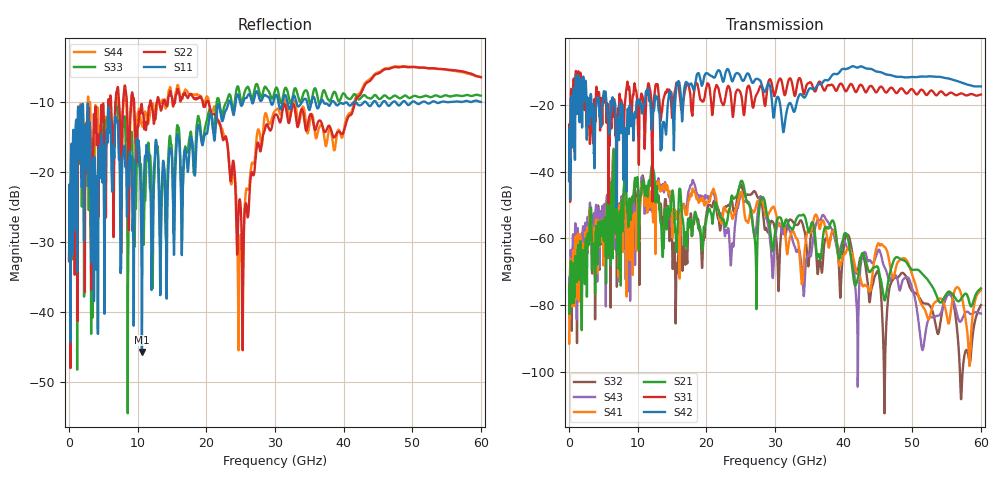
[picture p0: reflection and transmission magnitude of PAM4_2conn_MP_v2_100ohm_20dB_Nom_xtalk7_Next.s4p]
! Info: Touchstone file created by Circ.  Input file=FAB50GbE_2conn_Midplane_Examax_Topo2_v2_100ohm_20dB_Nom.circ
# Hz S RI R 50
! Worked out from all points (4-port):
!   6000 points, 10 MHz to 60 GHz, reference 50 ohm
!   strongest paths, dB at 10 MHz, 15.01 GHz, 30.01 GHz, 45.01 GHz, 60 GHz:
!     S42: -42.6, -18.4, -20.8, -10.2, -14.6
!     S31: -42.8, -23.9, -17.0, -15.7, -17.0
!     S21: -75.8, -46.0, -58.2, -68.7, -74.9
!     S41: -88.9, -56.3, -51.5, -61.6, -75.4
!     S43: -77.4, -53.4, -60.7, -63.6, -82.4
!     S32: -81.8, -60.5, -57.4, -69.8, -79.9
!   lowest |S11| = -45.7 dB at 10.62 GHz (marker M1), VSWR 1.01, Z = 49.5 + j0.252 ohm
!   |S11| at or under -10 dB: start of sweep to 23.24 GHz; 38.68 GHz to 40.3 GHz (1.617 GHz wide, 4.09 % of centre); 41.79 GHz to 42.9 GHz (1.107 GHz wide, 2.61 % of centre)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
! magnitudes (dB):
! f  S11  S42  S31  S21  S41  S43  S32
! 10 MHz  -32.4  -42.6  -42.8  -75.8  -88.9  -77.4  -81.8
! 1.18 GHz  -34.3  -22.6  -20.1  -70.8  -69.6  -63.4  -76.7
! 10.62 GHz  -45.7  -22.4  -17.1  -44.2  -43.5  -41.7  -42.2
! 15.64 GHz  -16.3  -14.7  -13.5  -63.9  -52.1  -53.7  -70.2
! 24.87 GHz  -9.7  -11.1  -16.0  -44.0  -46.9  -47.9  -44.6
! 28.66 GHz  -9.0  -15.7  -19.3  -50.8  -53.2  -53.3  -56.9
! 60 GHz  -9.9  -14.6  -17.0  -74.9  -75.4  -82.4  -79.9
